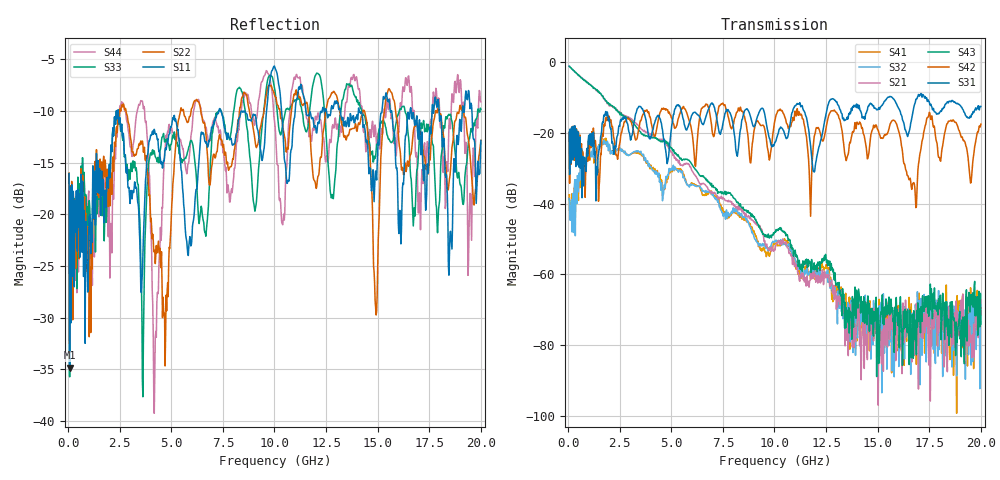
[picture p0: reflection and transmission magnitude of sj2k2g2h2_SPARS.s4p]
! FILE: E:\users\goganessyan\GBX_Backplane\FR408_backplane\1m_OUTBOUND_TRU\sj2k2g2h2_SPARS.s4p
# MHZ S RI R 50.00
! FREQ  S11  S12  S13  S14
!  S21  S22  S23  S24
!  S31  S32  S33  S34
!  S41  S42  S43  S44
!  REAL  IMAG  REAL  IMAG  REAL  IMAG  REAL  IMAG
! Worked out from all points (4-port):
!   799 points, 50 MHz to 20 GHz, reference 50 ohm
!   strongest paths, dB at 50 MHz, 5.025 GHz, 10.03 GHz, 15.03 GHz, 20 GHz:
!     S31: -19.7, -17.8, -22.6, -13.3, -12.5
!     S42: -19.9, -15.8, -16.3, -19.2, -17.5
!     S43: -1.1, -24.3, -48.0, -69.5, -74.1
!     S21: -1.1, -25.5, -53.1, -97.1, -67.4
!     S32: -38.6, -29.9, -50.5, -76.5, -68.6
!     S41: -37.5, -30.5, -51.4, -70.7, -71.5
!   lowest |S11| = -34.9 dB at 75 MHz (marker M1), VSWR 1.04, Z = 51.8 - j0.29 ohm
!   |S11| at or under -10 dB: start of sweep to 2.34 GHz; 2.429 GHz to 7.306 GHz (4.877 GHz wide, 100 % of centre); 14.1 GHz to 15.21 GHz (1.113 GHz wide, 7.6 % of centre)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
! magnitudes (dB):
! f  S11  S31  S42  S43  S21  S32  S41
! 50 MHz  -16.1  -19.7  -19.9  -1.1  -1.1  -38.6  -37.5
! 75 MHz  -34.9  -31.7  -34.2  -1.1  -1.1  -42.0  -42.0
! 3.45 GHz  -21.4  -12.5  -18.2  -19.4  -18.3  -25.3  -25.5
! 4.2 GHz  -12.0  -17.1  -21.0  -21.3  -21.1  -30.8  -30.1
! 4.875 GHz  -12.3  -26.5  -14.4  -23.7  -24.4  -30.9  -31.5
! 13.85 GHz  -11.1  -12.1  -19.5  -67.0  -80.7  -74.4  -70.9
! 20 GHz  -12.8  -12.5  -17.5  -74.1  -67.4  -68.6  -71.5
